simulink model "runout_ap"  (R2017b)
settings: Solver=VariableStepAuto  StartTime=0.0  StopTime=10.0  RelTol=1e-3

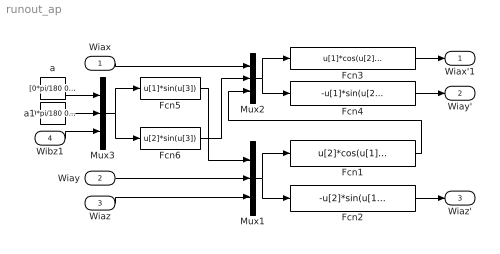
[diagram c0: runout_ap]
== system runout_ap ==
  Wiax : Inport
  Wiay : Inport  Port=2
  Wiaz : Inport  Port=3
  Wibz1 : Inport  Port=4
  Fcn1 : Fcn  Expr=u[2]*cos(u[1])+u[3]*sin(u[1])
  Fcn2 : Fcn  Expr=-u[2]*sin(u[1])+u[3]*cos(u[1])
  Fcn3 : Fcn  Expr=u[1]*cos(u[2])+u[3]*sin(u[2])
  Fcn4 : Fcn  Expr=-u[1]*sin(u[2])+u[3]*cos(u[2])
  Fcn5 : Fcn  Expr=u[1]*sin(u[3])
  Fcn6 : Fcn  Expr=u[2]*sin(u[3])
  Mux1 : Mux  Inputs=3
  Mux2 : Mux  Inputs=3
  Mux3 : Mux  Inputs=3
  a : Constant  Value=[0*pi/180 0*pi/180 0*pi/180]'
  a1 : Constant  Value=[0*pi/180 0*pi/180 0*pi/180]'
  Wiax'1 : Outport
  Wiay' : Outport  Port=2
  Wiaz' : Outport  Port=3
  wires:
  Fcn1/1 -> Mux2/3
  Mux1/1 -> Fcn2/1, Fcn1/1
  Fcn4/1 -> Wiay'/1
  Wiaz/1 -> Mux1/3
  Wiay/1 -> Mux1/2
  Wiax/1 -> Mux2/1
  Mux2/1 -> Fcn4/1, Fcn3/1
  Fcn2/1 -> Wiaz'/1
  Fcn3/1 -> Wiax'1/1
  a1/1 -> Mux3/2
  a/1 -> Mux3/1
  Wibz1/1 -> Mux3/3
  Fcn6/1 -> Mux2/2
  Mux3/1 -> Fcn6/1, Fcn5/1
  Fcn5/1 -> Mux1/1
